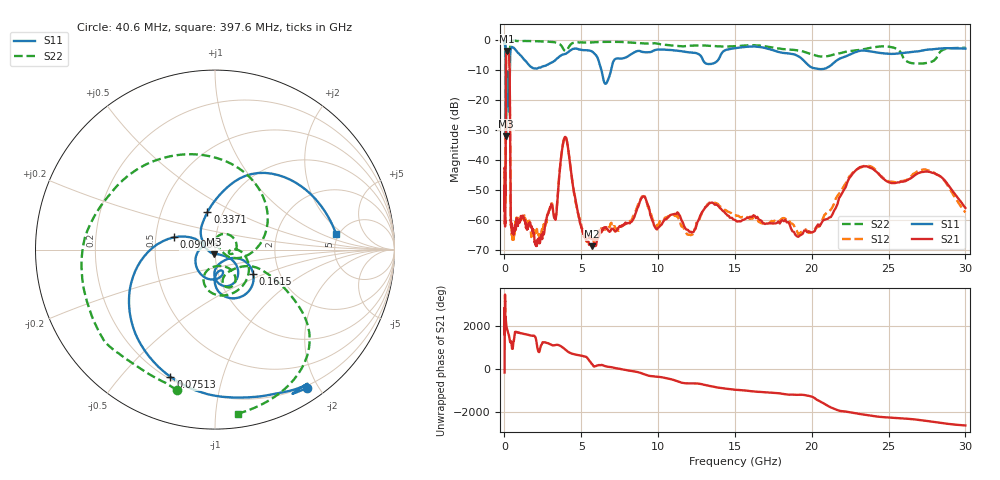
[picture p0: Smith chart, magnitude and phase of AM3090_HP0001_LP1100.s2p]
! Date/Time: Thu, Feb 28, 2019 1:54 PM
! Network Analyzer: Agilent Technologies E8364B Rev: A.07.50.67
! Sweep from 0.010 to 30.000 GHz, 1601 Points, Sweep Type: LOG
! Power Supply: 5.023 V, 0.002 A
# Hz S DB R 50
!freq MagS11 AngS11 MagS21 AngS21 MagS12 AngS12 MagS22 AngS22
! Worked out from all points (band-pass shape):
!   1601 points, 10 MHz to 30 GHz, reference 50 ohm
!   highest |S21| = -3.59 dB at 155.2 MHz (marker M1); lowest = -68.9 dB at 5.697 GHz (marker M2)
!   |S21| within 3 dB of the highest: 100.8 MHz to 319.8 MHz (219 MHz wide, 104 % of centre)
!   lowest |S11| = -32.1 dB at 98.93 MHz (marker M3), VSWR 1.05, Z = 49.5 - j2.43 ohm
!   |S11| at or under -10 dB: 89.6 MHz to 349.3 MHz (259.7 MHz wide, 118 % of centre); 6.308 GHz to 6.937 GHz (628.9 MHz wide, 9.5 % of centre)
!   |S22| runs from -33.4 to -0.1 dB; largest |S21 - S12| = 0.012
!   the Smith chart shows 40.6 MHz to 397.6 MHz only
!   S11 on the Smith chart (normalised r, x): 40.6 MHz: 0.17, -1.85; 75.13 MHz: 0.21, -0.69; 90.86 MHz: 0.62, +0.09; 161.5 MHz: 1.47, -0.42; 337.1 MHz: 0.85, +0.37; 397.6 MHz: 4.74, +1.54
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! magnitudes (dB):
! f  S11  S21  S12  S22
! 10 MHz  -0.3  -42.8  -46.1  -0.7
! 38.04 MHz  -0.5  -61.9  -60.9  -1.6
! 40.6 MHz  -0.7  -60.4  -59.4  -1.8
! 75.13 MHz  -2.5  -44.8  -44.4  -4.5
! 90.86 MHz  -12.4  -14.2  -14.1  -12.7
! 98.93 MHz  -32.1  -7.2  -7.2  -32.7
! 114.4 MHz  -13.5  -4.8  -4.8  -19.3
! 144.7 MHz  -19.7  -3.6  -3.6  -21.4
! 155.2 MHz  -13.8  -3.6  -3.6  -17.0
! 161.5 MHz  -12.0  -3.6  -3.6  -14.9
! 303.5 MHz  -24.0  -5.3  -5.3  -16.6
! 337.1 MHz  -13.5  -10.0  -10.0  -8.4
! 397.6 MHz  -3.3  -54.6  -55.0  -0.7
! 550.5 MHz  -2.5  -62.9  -66.0  -0.2
! 2.084 GHz  -9.5  -68.7  -64.1  -0.4
! 3.302 GHz  -6.7  -59.8  -59.1  -0.8
! 3.953 GHz  -4.7  -32.3  -32.3  -3.6
! 5.697 GHz  -3.8  -68.9  -66.5  -0.8
! 7.926 GHz  -5.7  -61.3  -61.2  -0.7
! 19.51 GHz  -7.0  -63.6  -63.7  -3.9
! 23.36 GHz  -3.5  -42.2  -42.1  -3.1
! 30 GHz  -2.9  -56.1  -57.6  -2.6
